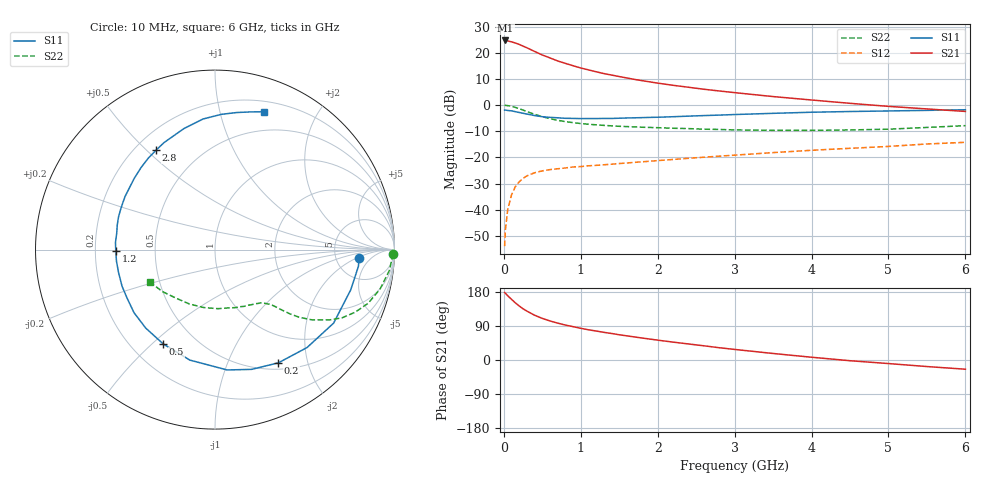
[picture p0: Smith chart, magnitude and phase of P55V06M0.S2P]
! SIEMENS Small Signal Semiconductors
! BFP183
! Si NPN RF Bipolar Junction Transistor in SOT143
! VCE = 5 V  IC = 6 mA
! Common Emitter S-Parameters:  March  1996
# GHz  S  MA  R  50
!  f  S11  S21  S12  S22
! GHz  MAG  ANG  MAG  ANG  MAG  ANG  MAG  ANG
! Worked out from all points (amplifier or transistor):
!   36 points, 10 MHz to 6 GHz, reference 50 ohm
!   highest |S21| = 24.7 dB at 20 MHz (marker M1)
!   |S21| within 3 dB of that: start of sweep to 313.9 MHz
!   unconditionally stable (mu >= 1): 1.496 GHz to 5.653 GHz
!   at 250 MHz: K = 0.23, MSG = 25.3 dB, |S12| = -28.0 dB
!   at 1.4 GHz: K = 0.97, MSG = 17.1 dB, |S12| = -22.6 dB
!   at 6 GHz: K = 0.95, MSG = 5.9 dB, |S12| = -14.2 dB
!   lowest NFmin = 1.20 dB at 450 MHz
!   S11 on the Smith chart (normalised r, x): 10 MHz: 8.59, -2.24; 200 MHz: 0.58, -1.54; 500 MHz: 0.33, -0.54; 1.2 GHz: 0.29, -0.01; 2.8 GHz: 0.28, +0.54; 6 GHz: 0.30, +1.37
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0.01  0.8035 -3.3  17.11 178.0  0.002 82.1  0.9912 -1.4
0.02  0.8046 -6.6  17.27 176.2  0.0041 88.0  0.988 -2.8
0.05  0.7888 -16.5  16.91 169.7  0.0099 84.2  0.9781 -6.9
0.1  0.7775 -31.8  16.23 160.0  0.0192 74.2  0.9458 -13.4
0.15  0.7488 -46.8  15.44 150.7  0.0276 66.5  0.9044 -19.3
0.2  0.7229 -60.8  14.51 142.5  0.0341 60.8  0.8549 -24.1
0.25  0.6977 -73.0  13.44 135.1  0.0396 55.8  0.8038 -28.2
0.3  0.6741 -84.2  12.5 129.0  0.0443 52.0  0.7509 -31.4
0.4  0.6314 -102.8  10.63 118.1  0.0508 45.2  0.6679 -35.9
0.5  0.5998 -118.7  9.096 109.8  0.0552 40.5  0.6013 -38.8
0.6  0.5832 -131.5  8.001 103.0  0.0583 38.0  0.5502 -40.6
0.7  0.5719 -142.1  6.999 97.3  0.0605 36.3  0.5113 -41.8
0.9  0.5566 -158.5  5.669 88.0  0.0655 34.2  0.4623 -43.4
1.1  0.5527 -173.2  4.723 79.7  0.069 33.6  0.4299 -45.1
1.2  0.5529 -179.1  4.344 76.5  0.0703 33.2  0.4199 -46.0
1.7  0.5718 156.7  3.101 60.8  0.0803 33.9  0.3828 -51.7
2.2  0.5998 138.7  2.392 47.2  0.0913 34.4  0.3609 -59.2
2.8  0.644 120.6  1.865 32.4  0.1055 33.7  0.3424 -70.9
3.5  0.6962 104.4  1.457 17.2  0.1234 31.9  0.3295 -87.1
4.5  0.7544 87.3  1.082 -1.9  0.1491 26.9  0.3349 -115.2
5.5  0.7932 75.3  0.845 -17.3  0.1803 21.6  0.3742 -141.2
6  0.815 70.4  0.757 -24.3  0.1941 17.7  0.4048 -153.2
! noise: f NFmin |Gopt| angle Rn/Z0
0.45  1.2  0.21  41  0.24
0.9  1.25  0.24  101  0.21
1.8  2  0.32  175  0.14
